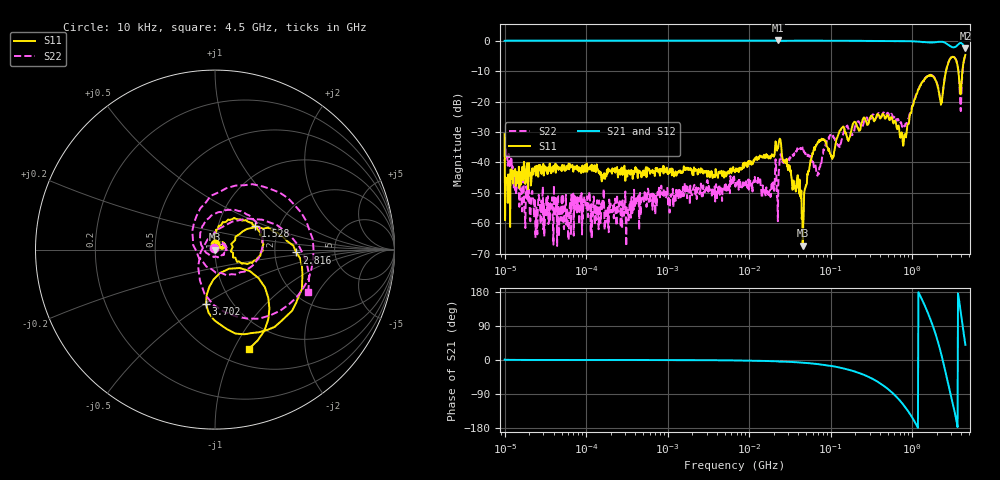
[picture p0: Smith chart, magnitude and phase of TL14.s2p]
!Siglent Technologies,SNA5004A,SNA5XCED5R0097,V1.0.0.2.10.R9
!Date: 2024-11-24 17:48:05
!Data & Calibration Information:
!Freq	S11:F2(ON)	S21:F2(ON)	S12:F2(ON)	S22:F2(ON)
# Hz S RI R 50
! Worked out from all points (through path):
!   1001 points, 10 kHz to 4.5 GHz, reference 50 ohm
!   highest |S21| = 0.11 dB at 22.8 MHz (marker M1); lowest = -2.4 dB at 4.5 GHz (marker M2)
!   group delay of S21, straight-line fit = 419 ps
!   lowest |S11| = -67.3 dB at 45.46 MHz (marker M3), VSWR 1.00, Z = 50 - j0.000803 ohm
!   |S11| at or under -10 dB: start of sweep to 2.6 GHz; 3.693 GHz to 4.133 GHz (440.5 MHz wide, 11.3 % of centre)
!   |S22| runs from -67.5 to -4.9 dB; largest |S21 - S12| = 0.025
!   S11 on the Smith chart (normalised r, x): 10 kHz: 1.00, +0.06; 1.528 GHz: 1.51, +0.42; 2.816 GHz: 2.65, -0.11; 3.702 GHz: 0.76, -0.51; 4.5 GHz: 0.68, -1.15
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10000  0.00215 0.0291  1.001 0.0152  0.9978 0.0187  -0.00385 0.00978
10953.99  0.00205 0.000718  1.006 0.00418  0.9981 0.00475  0.00187 0.00866
23920.22  0.00859 0.00106  1.008 0.00164  1 -0.00056  0.000242 0.000524
87919.76  0.00704 0.00072  1.008 0.000173  1.001 -0.00208  0.0024 -0.00203
772988.4  0.00657 0.00202  1.007 -0.00206  1.001 -0.00435  0.00182 -0.00217
6708204  0.00307 0.00619  1.005 -0.0182  0.9965 -0.0213  -0.0026 -0.00367
2.280385e7  -0.0101 0.0152  1.01 -0.067  1.002 -0.0661  -0.00132 0.00387
4.54599e7  0.000432 -8.03e-06  0.9984 -0.1245  0.9869 -0.1229  0.00127 0.0176
5.897837e7  0.00856 0.00901  0.9883 -0.1601  0.981 -0.1595  -0.00492 0.0101
7.076813e7  0.00737 0.0201  0.985 -0.1905  0.9759 -0.1891  0.000274 0.00666
2.343869e8  0.0251 0.0297  0.8075 -0.5834  0.8023 -0.5765  0.0223 0.0329
5.185364e8  0.0463 0.0237  0.1951 -0.9704  0.1986 -0.9629  0.0605 -0.00245
8.072136e8  0.0165 0.0236  -0.5252 -0.8342  -0.5181 -0.8322  -0.0164 -0.0355
1.162193e9  0.0353 0.1375  -0.9699 -0.062  -0.9651 -0.0671  -0.0703 0.1307
1.527552e9  0.2235 0.1294  -0.592 0.7348  -0.5939 0.7253  0.164 0.2047
1.881253e9  0.2338 -0.0508  0.2123 0.918  0.2021 0.9142  0.2443 -0.0464
2.257315e9  0.0883 -0.00982  0.9162 0.3053  0.907 0.3111  -0.0689 -0.0663
2.816416e9  0.4528 -0.0159  0.2975 -0.7966  0.3049 -0.7881  0.3052 0.3394
3.249991e9  0.3322 -0.4309  -0.4817 -0.6112  -0.4701 -0.6169  0.5192 -0.168
3.701812e9  -0.0499 -0.3034  -0.8603 0.1764  -0.8579 0.1609  -0.00865 -0.308
4.054962e9  0.1939 -0.1195  -0.2781 0.8621  -0.2951 0.8511  0.0956 0.1556
4.5e9  0.1885 -0.5535  0.5821 0.4896  0.5669 0.4987  0.5199 -0.2361
